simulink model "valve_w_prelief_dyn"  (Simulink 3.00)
settings: Solver=ode45  StartTime=0.0  StopTime=10.0  RelTol=1e-3
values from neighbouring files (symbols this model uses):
  dt = tfinal/N    (= 0.02)    [demo_trench.m]
  prelief = 2250    [backhoesim.m]
  QP = 33.11    [backhoesim.m]
  T = 0.001    [startup.m]
undefined symbols (not defined in the file or in its folder): den, K1, kd, Kr, num, td, wn, zeta
libraries: simulink3 x1

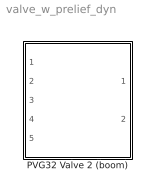
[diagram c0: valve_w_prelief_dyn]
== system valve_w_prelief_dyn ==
  PVG32 Valve 2 (boom) : Subsystem

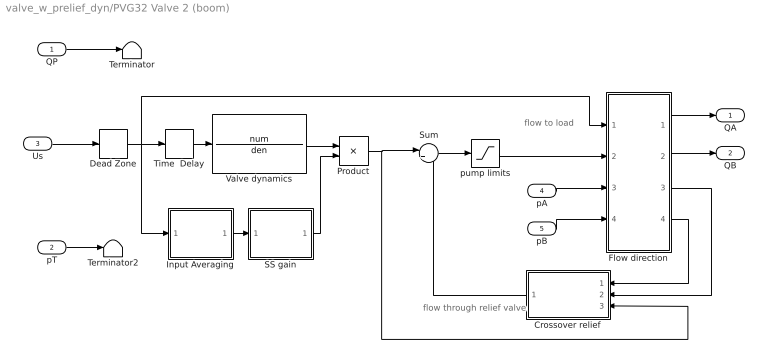
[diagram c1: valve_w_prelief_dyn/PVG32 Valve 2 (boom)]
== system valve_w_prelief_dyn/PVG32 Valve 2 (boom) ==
  note: flow to load
  note: flow through relief valve
  QP : Inport  Port=1  PortWidth=-1  SampleTime=-1  DataType=auto
  pT : Inport  Port=2  PortWidth=-1  SampleTime=-1  DataType=auto
  Us : Inport  Port=3  PortWidth=-1  SampleTime=-1  DataType=auto
  pA : Inport  Port=4  PortWidth=-1  SampleTime=-1  DataType=auto
  pB : Inport  Port=5  PortWidth=-1  SampleTime=-1  DataType=auto
  Crossover relief : Subsystem  Orientation=left
  Dead Zone : DeadZone  LowerValue=-.5  UpperValue=.5
  Flow direction : Subsystem
  Input Averaging : Subsystem
  Product : Product  Inputs=2  SaturateOnIntegerOverflow=on
  SS gain : Subsystem
  Sum : Sum  Inputs=|+-  SaturateOnIntegerOverflow=on
  Terminator : Terminator
  Terminator2 : Terminator
  Time  Delay : TransportDelay  DelayTime=td  InitialInput=0  BufferSize=2048
  Valve dynamics : TransferFcn  Numerator=num  Denominator=den
  pump limits : Saturate  UpperLimit=QP  LowerLimit=-QP
  QA : Outport  Port=1
  QB : Outport  Port=2
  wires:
  pB/1 -> Flow direction/4(pB)
  pA/1 -> Flow direction/3(pA)
  pT/1 -> Terminator2/1
  Time  Delay/1 -> Valve dynamics/1
  Us/1 -> Dead Zone/1
  Dead Zone/1 -> Time  Delay/1, Flow direction/1(Us), Input Averaging/1(Us)
  Valve dynamics/1 -> Product/1
  Input Averaging/1(Ubar) -> SS gain/1(Ubar)
  SS gain/1(Kv) -> Product/2
  Product/1 -> Sum/1, Crossover relief/3(Q)
  Crossover relief/1(Qrelief) -> Sum/2
  QP/1 -> Terminator/1
  Sum/1 -> pump limits/1
  Flow direction/1(QA) -> QA/1
  Flow direction/2(QB) -> QB/1
  Flow direction/4(pR) -> Crossover relief/1(pR)
  Flow direction/3(pL) -> Crossover relief/2(pL)
  pump limits/1 -> Flow direction/2(Q)

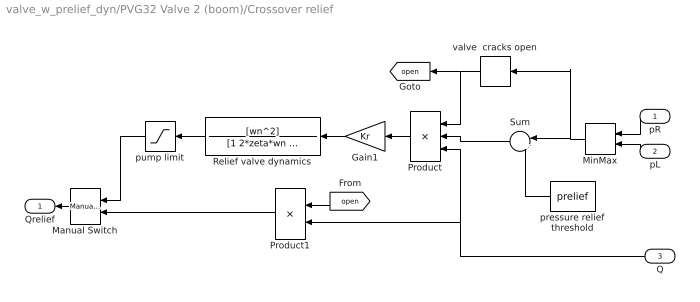
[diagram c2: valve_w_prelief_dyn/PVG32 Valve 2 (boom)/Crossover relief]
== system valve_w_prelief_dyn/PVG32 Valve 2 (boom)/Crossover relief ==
  pR : Inport  Orientation=left  Port=1  PortWidth=-1  SampleTime=-1  DataType=auto
  pL : Inport  Orientation=left  Port=2  PortWidth=-1  SampleTime=-1  DataType=auto
  Q : Inport  Orientation=left  Port=3  PortWidth=-1  SampleTime=-1  DataType=auto
  Gain1 : Gain  Orientation=left  Gain=Kr  SaturateOnIntegerOverflow=on
  Manual Switch : simulink3/Nonlinear/Manual Switch  Orientation=left  sw=0  action=0
  MinMax : MinMax  Orientation=left  Function=max  Inputs=2
  Product : Product  Orientation=left  Inputs=3  SaturateOnIntegerOverflow=on
  Product1 : Product  Orientation=left  Inputs=2  SaturateOnIntegerOverflow=on
  Relief valve dynamics : TransferFcn  Orientation=left  Numerator=[wn^2]  Denominator=[1 2*zeta*wn wn^2]
  Sum : Sum  Orientation=left  Inputs=|+-  SaturateOnIntegerOverflow=on
  pressure relief threshold : Constant  Orientation=left  Value=prelief
  pump limit : Saturate  Orientation=left  UpperLimit=QP  LowerLimit=0
  valve  cracks open : Relay  Orientation=left  OnSwitchValue=prelief  OffSwitchValue=prelief  OnOutputValue=1  OffOutputValue=0
  Qrelief : Outport  Orientation=left  Port=1
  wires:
  Manual Switch/1 -> Qrelief/1
  Product/1 -> Gain1/1
  Gain1/1 -> Relief valve dynamics/1
  Relief valve dynamics/1 -> pump limit/1
  Sum/1 -> Product/2
  pressure relief threshold/1 -> Sum/2
  pR/1 -> MinMax/1
  pL/1 -> MinMax/2
  MinMax/1 -> Sum/1, valve  cracks open/1
  pump limit/1 -> Manual Switch/1
  Product1/1 -> Manual Switch/2
  Q/1 -> Product/3, Product1/2
  [open] -> Product1/1
  valve  cracks open/1 -> Product/1, [open]

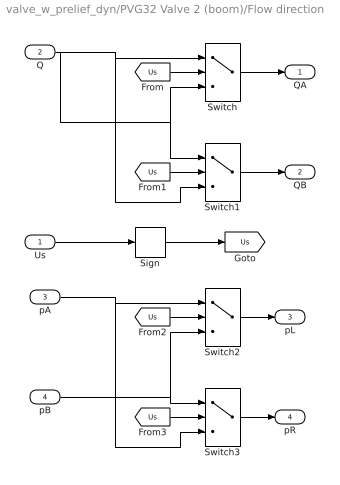
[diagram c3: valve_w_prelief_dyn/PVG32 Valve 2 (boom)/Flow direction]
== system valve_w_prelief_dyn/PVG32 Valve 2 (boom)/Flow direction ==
  Us : Inport  Port=1  PortWidth=-1  SampleTime=-1  DataType=auto
  Q : Inport  Port=2  PortWidth=-1  SampleTime=-1  DataType=auto
  pA : Inport  Port=3  PortWidth=-1  SampleTime=-1  DataType=auto
  pB : Inport  Port=4  PortWidth=-1  SampleTime=-1  DataType=auto
  Sign : Signum
  Switch{,1..3} (4 alike) : Switch  Threshold=0
  QA : Outport  Port=1
  QB : Outport  Port=2
  pL : Outport  Port=3
  pR : Outport  Port=4
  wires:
  [Us] -> Switch/2
  [Us] -> Switch1/2
  Switch1/1 -> QB/1
  Switch/1 -> QA/1
  Us/1 -> Sign/1
  Sign/1 -> [Us]
  pA/1 -> Switch2/1, Switch3/3
  [Us] -> Switch2/2
  [Us] -> Switch3/2
  pB/1 -> Switch2/3, Switch3/1
  Switch2/1 -> pL/1
  Switch3/1 -> pR/1
  Q/1 -> Switch1/3, Switch/1, Switch1/1, Switch/3

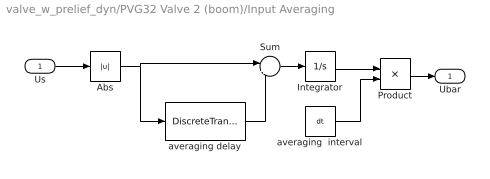
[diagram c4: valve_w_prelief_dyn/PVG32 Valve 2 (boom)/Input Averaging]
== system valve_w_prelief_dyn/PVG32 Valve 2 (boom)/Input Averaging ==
  Us : Inport  Port=1  PortWidth=-1  SampleTime=-1  DataType=auto
  Abs : Abs
  Integrator : Integrator  ExternalReset=none  InitialConditionSource=internal  InitialCondition=0  LimitOutput=off  UpperSaturationLimit=inf  LowerSaturationLimit=-inf  ShowSaturationPort=off  ShowStatePort=off  AbsoluteTolerance=auto
  Product : Product  Inputs=*/  SaturateOnIntegerOverflow=on
  Sum : Sum  Inputs=|+-  SaturateOnIntegerOverflow=on
  averaging  interval : Constant  Value=dt
  averaging delay : DiscreteTransferFcn  Numerator=[1]  Denominator=[1 zeros(1,kd)]  SampleTime=T
  Ubar : Outport  Port=1
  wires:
  averaging  interval/1 -> Product/2
  Us/1 -> Abs/1
  Abs/1 -> averaging delay/1, Sum/1
  Product/1 -> Ubar/1
  Sum/1 -> Integrator/1
  averaging delay/1 -> Sum/2
  Integrator/1 -> Product/1

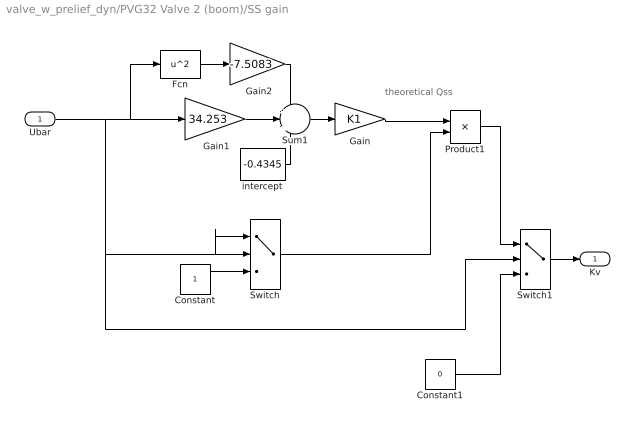
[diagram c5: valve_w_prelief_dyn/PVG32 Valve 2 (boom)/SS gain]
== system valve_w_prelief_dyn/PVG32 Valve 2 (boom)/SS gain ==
  note: theoretical Qss
  Ubar : Inport  Port=1  PortWidth=-1  SampleTime=-1  DataType=auto
  " Gain1" : Gain  Gain=34.253  SaturateOnIntegerOverflow=on
  " Gain2" : Gain  Gain=-7.5083  SaturateOnIntegerOverflow=on
  Constant : Constant  Value=1
  Constant1 : Constant  Value=0
  Fcn : Fcn  Expr=u^2
  Gain : Gain  Gain=K1  SaturateOnIntegerOverflow=on
  Product1 : Product  Inputs=*/  SaturateOnIntegerOverflow=on
  Sum1 : Sum  Inputs=+|+|+  SaturateOnIntegerOverflow=on
  Switch : Switch  Threshold=0.001
  Switch1 : Switch  Threshold=0
  intercept : Constant  Value=-0.4345
  Kv : Outport  Port=1
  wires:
  " Gain2"/1 -> Sum1/1
  " Gain1"/1 -> Sum1/2
  intercept/1 -> Sum1/3
  Fcn/1 -> " Gain2"/1
  Constant/1 -> Switch/3
  Switch/1 -> Product1/2
  Product1/1 -> Switch1/1
  Switch1/1 -> Kv/1
  Constant1/1 -> Switch1/3
  Gain/1 -> Product1/1
  Sum1/1 -> Gain/1
  Ubar/1 -> " Gain1"/1, Fcn/1, Switch/2, Switch/1, Switch1/2
